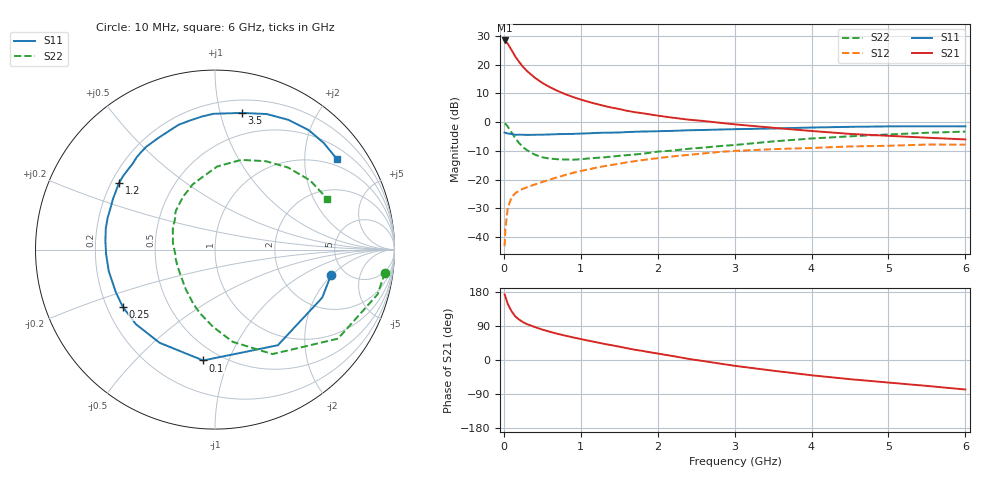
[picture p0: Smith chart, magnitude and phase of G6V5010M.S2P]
! SIEMENS Small Signal Semiconductors
! BFG193
! Si NPN RF Bipolar Junction Transistor in SOT223
! VCE = 0.5 V  IC = 10 mA
! Common Emitter S-Parameters:  August  1996
# GHz  S  MA  R  50
!  f  S11  S21  S12  S22
! GHz  MAG  ANG  MAG  ANG  MAG  ANG  MAG  ANG
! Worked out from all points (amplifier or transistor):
!   36 points, 10 MHz to 6 GHz, reference 50 ohm
!   highest |S21| = 28.4 dB at 10 MHz (marker M1)
!   |S21| within 3 dB of that: start of sweep to 92.9 MHz
!   unconditionally stable (mu >= 1): 764.9 MHz to 4.709 GHz; 5.624 GHz to end of sweep
!   at 250 MHz: K = 0.56, MSG = 21.2 dB, |S12| = -23.1 dB
!   at 1.4 GHz: K = 1.10, MAG = 8.0 dB, |S12| = -14.9 dB
!   at 6 GHz: K = 1.01, MAG = 0.3 dB, |S12| = -7.8 dB
!   S11 on the Smith chart (normalised r, x): 10 MHz: 3.90, -1.94; 100 MHz: 0.40, -0.81; 250 MHz: 0.27, -0.27; 1.2 GHz: 0.23, +0.30; 3.5 GHz: 0.31, +1.17; 6 GHz: 0.79, +2.82
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0.01  0.6619 -12.2  26.37 173.1  0.007 86.2  0.9558 -7.7
0.02  0.6547 -24.1  25.87 167.2  0.0138 80.5  0.9395 -15.4
0.05  0.6376 -56.7  23.2 148.5  0.032 64.5  0.8461 -35.9
0.1  0.6212 -96.1  18.01 128.7  0.0496 51.9  0.6643 -61.2
0.15  0.604 -120.7  13.75 114.8  0.0584 43.9  0.5228 -79.2
0.2  0.6057 -136.6  11.11 106.5  0.0649 41.2  0.4319 -91.2
0.25  0.6048 -148.1  9.154 99.8  0.0696 39.9  0.367 -102.7
0.3  0.6015 -156.6  7.792 94.8  0.0739 39.9  0.3272 -111.4
0.4  0.604 -168.5  5.974 87.1  0.0824 40.2  0.2738 -126.6
0.5  0.6072 -177.5  4.814 80.3  0.0911 41.2  0.2451 -139.0
0.6  0.6128 175.3  4.055 74.5  0.101 41.8  0.2326 -149.2
0.7  0.6202 168.7  3.496 69.0  0.1107 42.1  0.2273 -158.4
0.8  0.6238 163.4  3.063 64.2  0.1211 41.5  0.2248 -166.9
1.1  0.6406 149.7  2.259 51.0  0.1513 39.3  0.2342 174.1
1.2  0.6514 145.1  2.084 47.0  0.1618 38.3  0.2399 168.4
1.7  0.6813 127.2  1.496 27.1  0.2099 30.0  0.2746 145.5
2.2  0.7074 111.8  1.196 10.3  0.2546 19.4  0.3219 128.4
2.8  0.7453 95.5  0.98 -9.2  0.3039 6.3  0.3841 108.9
3.5  0.7764 78.8  0.8 -28.2  0.34 -10.6  0.4634 88.4
4.5  0.8305 60.5  0.626 -50.6  0.379 -29.0  0.5682 60.1
5.5  0.8485 44.4  0.538 -68.4  0.4087 -50.6  0.6554 36.0
6  0.8462 36.6  0.502 -77.9  0.407 -63.0  0.6868 24.3
